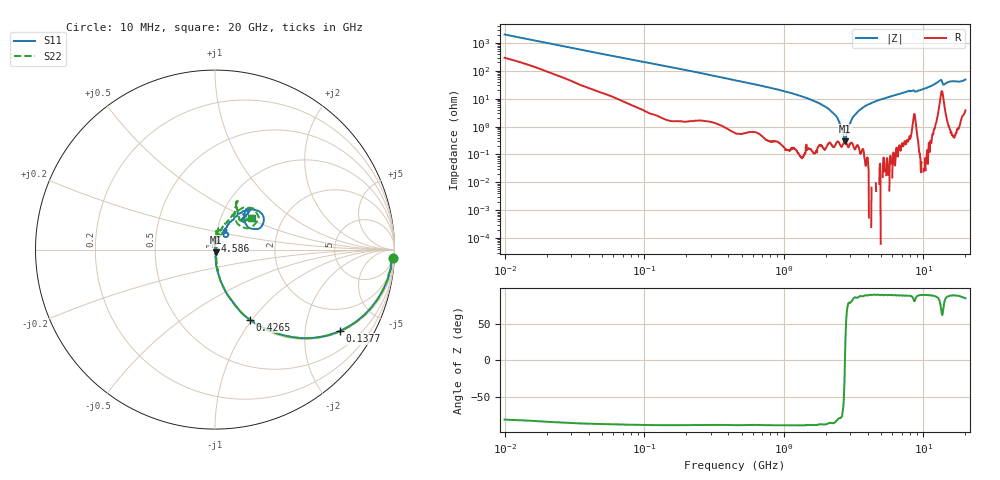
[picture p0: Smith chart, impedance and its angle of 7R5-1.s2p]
!Keysight Technologies,P5008B,MY61100088,A.16.20.02
!Date: Monday, May 27, 2024 16:40:56
!Correction: S11(C* 2-Port  )
!S21(C* 2-Port  )
!S12(C* 2-Port  )
!S22(C* 2-Port  )
!S2P File: Measurements: S11, S21, S12, S22:Log Frequency Sweep
# Hz S  dB  R 50
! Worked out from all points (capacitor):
!   1601 points, 10 MHz to 20 GHz, reference 50 ohm
!   read as one part in series: C = 8.01 pF near 10.39 MHz
!   lowest |Z| = 295 mohm at 2.746 GHz (marker M1)
!   series resonance near 2.743 GHz, so ESL is about 420 pH
!   S11 on the Smith chart (normalised r, x): 10 MHz: 5, -40; 137.7 MHz: 1.04, -3.04; 426.5 MHz: 1.01, -0.98; 4.586 GHz: 0.99, +0.10; 20 GHz: 1.41, +0.53
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1e7  -0.05 -2.8  -26.14 78.8  -26.16 78.8  -0.08 -2.8
3.555162e7  -0.21 -9.9  -15.24 77.0  -15.24 77.0  -0.22 -10.0
1.263918e8  -1.42 -31.0  -5.79 58.2  -5.80 58.2  -1.41 -31.1
1.376751e8  -1.61 -33.1  -5.28 56.2  -5.29 56.2  -1.60 -33.2
4.264652e8  -7.20 -63.5  -0.98 25.7  -0.99 25.7  -7.19 -63.7
4.472136e8  -7.52 -64.6  -0.90 24.6  -0.91 24.7  -7.52 -64.8
1.589917e9  -20.42 -84.8  -0.04 4.7  -0.05 4.7  -20.30 -83.3
2.336087e9  -28.25 -85.8  -0.00 0.7  -0.01 0.7  -27.86 -80.5
2.745591e9  -35.94 -76.2  0.00 -0.9  -0.01 -0.9  -35.26 -64.5
2.976524e9  -41.99 -65.9  0.01 -1.8  -0.00 -1.8  -41.45 -36.4
3.166141e9  -49.88 70.9  0.01 -2.4  -0.00 -2.4  -40.85 39.3
3.44879e9  -37.37 90.6  0.01 -3.3  -0.00 -3.3  -33.86 61.5
3.633803e9  -34.09 92.1  0.01 -3.9  -0.00 -3.9  -31.40 67.1
4.586226e9  -26.22 92.2  0.01 -6.6  -0.00 -6.6  -25.63 72.0
5.652411e9  -23.14 78.5  -0.00 -9.3  -0.01 -9.3  -23.23 81.5
7.697294e9  -18.56 60.8  -0.04 -14.4  -0.05 -14.5  -18.79 82.8
9.220141e9  -20.33 62.2  -0.03 -17.0  -0.04 -17.0  -20.28 77.2
1.304209e10  -10.27 46.9  -0.84 -30.0  -0.85 -30.0  -10.46 50.5
1.413906e10  -12.89 44.4  -0.60 -23.6  -0.61 -23.6  -13.61 57.3
1.569675e10  -10.36 50.5  -0.40 -29.8  -0.40 -29.8  -10.42 66.0
1.836088e10  -13.24 47.7  -0.26 -35.9  -0.27 -36.0  -13.38 51.0
2e10  -11.31 39.9  -0.59 -40.6  -0.60 -40.6  -11.44 41.1
